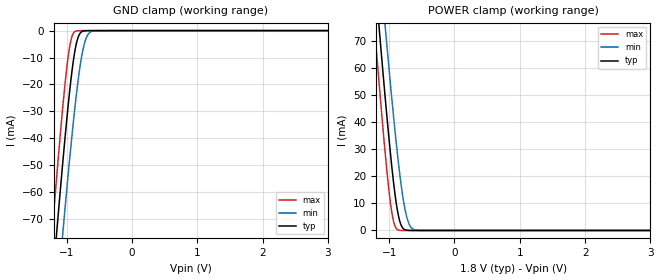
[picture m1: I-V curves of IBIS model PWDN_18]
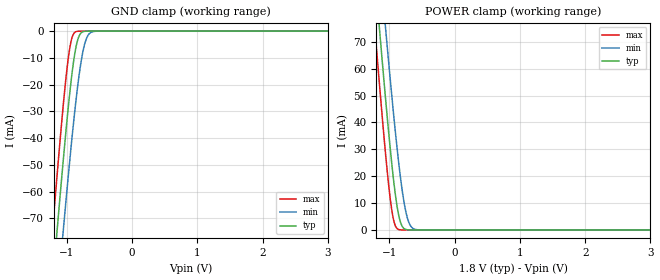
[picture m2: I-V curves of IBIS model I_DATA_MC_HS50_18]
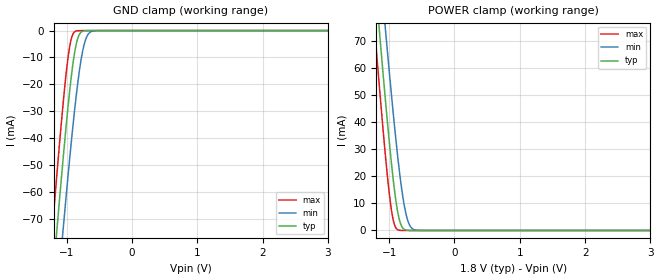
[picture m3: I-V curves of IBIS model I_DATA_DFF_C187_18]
| Texas Instruments Incorporated
| Low Power 1.8V FPD-Link (LVDS) Serializer
| Marketing part#   Voltage Range   Package-type   Temperature
| DS90C185SQE   1.71V - 1.89V   48-Pin LLP   -10 to 70C
| DS90C185SQ   1.71V - 1.89V   48-Pin LLP   -10 to 70C
| DS90C185SQX   1.71V - 1.89V   48-Pin LLP   -10 to 70C
[IBIS Ver]   4.0
[File name]   ds90c185.ibs
[File Rev]   1.0
[Date]   03/05/2012
[Source]   Model built from TISPICE simulations at:
   Texas Instruments Incorporated.
   WEBENCH DESIGN CENTER
   12500 TI Blvd
   Dallas, TX -75243
   For Support e-mail: elab_scm_ibis@list.ti.com
[Notes]   Rev 1.0: 03/05/2012
   - IBIS model generated from simulations from Spectre
   - ccomp is listed in numerical order and not by PVT case.
[Disclaimer] This product is designed as an aid for customers of Texas Instruments.
   No warranties, either expressed or implied, with respect to this third
   party software (if any) or with respect to its fitness for any
   particular purpose is claimed by Texas Instruments or the author. The
   software (if any) is provided solely on an "as is" basis. The entire
   risk as to its quality and performance is with the customer
[Copyright]   (C)Copyright 2012 Texas Instruments Incorporated.
   All rights reserved.
[Component]  DS90C185SQ
[Manufacturer]  Texas Instruments, Inc
[Package]   |48-pin LLP 6.0X6.0X0.8mm
|   typ   min   max
R_pkg   0   0   0
L_pkg   0   0   0
C_pkg   0   0   0
[Pin]   signal_name   model_name   R_pin   L_pin   C_pin
1   D9   I_DATA_DFF_C187_18
2   D10   I_DATA_DFF_C187_18
3   D11   I_DATA_DFF_C187_18
4   D12   I_DATA_DFF_C187_18
5   D13   I_DATA_DFF_C187_18
6   CLK   I_DATA_DFF_C187_18
7   D14   I_DATA_DFF_C187_18
8   D15   I_DATA_DFF_C187_18
9   D16   I_DATA_DFF_C187_18
10   D17   I_DATA_DFF_C187_18
11   D18   I_DATA_DFF_C187_18
12   D19   I_DATA_DFF_C187_18
13   VDDPLL   POWER
14   D20   I_DATA_DFF_C187_18
15   GND   GND
16   D21   I_DATA_DFF_C187_18
17   D22   I_DATA_DFF_C187_18
18   D23   I_DATA_DFF_C187_18
19   D24   I_DATA_DFF_C187_18
20   D25   I_DATA_DFF_C187_18
21   D26   I_DATA_DFF_C187_18
22   D27   I_DATA_DFF_C187_18
23   RFB   I_DATA_MC_HS50_18
24   GND   GND
25   VDDTX   POWER
26   18B_MODE   I_DATA_MC_HS50_18
27   TXOUT3P   LVDS_OUT
28   TXOUT3N   LVDS_OUT
29   TXCLKOUTP   LVDS_OUT
30   TXCLKOUTN   LVDS_OUT
31   TXOUT2P   LVDS_OUT
32   TXOUT2N   LVDS_OUT
33   TXOUT1P   LVDS_OUT
34   TXOUT1N   LVDS_OUT
35   TXOUT0P   LVDS_OUT
36   TXOUT0N   LVDS_OUT
37   PDB   PWDN_18
38   D0   I_DATA_DFF_C187_18
39   VOD_SEL   I_DATA_MC_HS50_18
40   D1   I_DATA_DFF_C187_18
41   D2   I_DATA_DFF_C187_18
42   D3   I_DATA_DFF_C187_18
43   D4   I_DATA_DFF_C187_18
44   D5   I_DATA_DFF_C187_18
45   D6   I_DATA_DFF_C187_18
46   D7   I_DATA_DFF_C187_18
47   D8   I_DATA_DFF_C187_18
48   VDD   POWER
49   DAP   GND
[Package Model] 48LLP_DS90C185
[Diff pin]  inv_pin  vdiff  tdelay_typ  tdelay_min  tdelay_max
27   28   0.0   0.0s   0.0s   0.0s
29   30   0.0   0.0s   0.0s   0.0s
31   32   0.0   0.0s   0.0s   0.0s
33   34   0.0   0.0s   0.0s   0.0s
35   36   0.0   0.0s   0.0s   0.0s
[Define Package Model]  48LLP_DS90C185
| AD# DS90C1855SQ-01 RevA at 6GHz
[Manufacturer]  Unknown
[OEM]  Unknown
[Description]  None
[Number Of Pins]  48
[Pin Numbers]
|Pin Num   Terminal Name
1   | L1:1
2   | L2:2
3   | L3:3
4   | L4:4
5   | L5:5
6   | L6:6
7   | L7:7
8   | L8:8
9   | L9:9
10   | L10:10
11   | L11:11
12   | L12:12
13   | L13:13
14   | L14:14
15   | L15:15
16   | L16:16
17   | L17:17
18   | L18:18
19   | L19:19
20   | L20:20
21   | L21:21
22   | L22:22
23   | L23:23
24   | L24:24
25   | L25:25
26   | L26:26
27   | L27:27
28   | L28:28
29   | L29:29
30   | L30:30
31   | L31:31
32   | L32:32
33   | L33:33
34   | L34:34
35   | L35:35
36   | L36:36
37   | L37:37
38   | L38:38
39   | L39:39
40   | L40:40
41   | L41:41
42   | L42:42
43   | L43:43
44   | L44:44
45   | L45:45
46   | L46:W50
47   | L47:47
48   | L48:48
[Model Data]
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[End Model Data]
[End Package Model]
| Models and submodels in the file (4): PWDN_18 (Input), I_DATA_MC_HS50_18 (Input), I_DATA_DFF_C187_18 (Input), LVDS_OUT (Output)
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[Model]   PWDN_18
Model_type   Input
Vinl = 0.63V
Vinh = 1.17V
|   typ   min   max
|   (nom)   (weak)   (fast)
C_comp   0.5928pF   0.5928pF   0.5928pF
[Voltage Range]   1.800V   1.710V   1.890V
[Temperature Range]   25.0   105.0   -40.0
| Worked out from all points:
|   GND clamp passes 1 mA (typ) near -0.79 V on its own axis
|   POWER clamp passes 1 mA (typ) near -0.79 V on its own axis
[GND Clamp]
|   Voltage   I(typ)   I(min)   I(max)
-1.8V     -270.9mA   -291mA     -255.6mA
-1.228V   -97.1mA    -122.7mA   -76.77mA
-1.201V   -89.21mA   -115mA     -68.71mA
-1.147V   -73.63mA   -99.73mA   -52.87mA
-1.055V   -48.06mA   -74.39mA   -27.51mA
-957.6mV  -23.54mA   -48.82mA   -6.663mA
-871.2mV  -7.328mA   -28.21mA   -335.2uA
-811.8mV  -1.781mA   -16.28mA   -25.67uA
-741.6mV  -161.6uA   -6.205mA   -6.921uA
-682.2mV  -20.1uA    -1.83mA    -5.854uA
-601.2mV  -4.02uA    -199.2uA   -5.127uA
3.595V    6.712uA    3.483uA    12.03uA
[POWER Clamp]
|   Voltage   I(typ)   I(min)   I(max)
-1.8V     270.2mA    290.2mA    254.8mA
-1.228V   96.77mA    122.3mA    76.49mA
-1.201V   88.9mA     114.6mA    68.45mA
-1.147V   73.36mA    99.39mA    52.65mA
-1.055V   47.86mA    74.11mA    27.37mA
-957.6mV  23.41mA    48.61mA    6.6mA
-871.2mV  7.262mA    28.06mA    325.8uA
-811.8mV  1.758mA    16.17mA    20.65uA
-741.6mV  156.5uA    6.146mA    2.661uA
-682.2mV  17.07uA    1.807mA    2.011uA
-601.2mV  1.608uA    195uA      1.824uA
3.595V    0A         0A         0A
[Model]   I_DATA_MC_HS50_18
Model_type   Input
Vinl = 0.63V
Vinh = 1.17V
|   typ   min   max
|   (nom)   (weak)   (fast)
C_comp   0.5928pF   0.5928pF   0.5928pF
[Voltage Range]   1.800V   1.710V   1.890V
[Temperature Range]   25.0   105.0   -40.0
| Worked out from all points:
|   GND clamp passes 1 mA (typ) near -0.79 V on its own axis
|   POWER clamp passes 1 mA (typ) near -0.79 V on its own axis
[GND Clamp]
|   Voltage   I(typ)   I(min)   I(max)
-1.8V     -271mA     -291mA     -255.6mA
-1.228V   -97.13mA   -122.7mA   -76.8mA
-1.201V   -89.24mA   -115mA     -68.74mA
-1.147V   -73.66mA   -99.76mA   -52.9mA
-1.055V   -48.09mA   -74.42mA   -27.54mA
-957.6mV  -23.57mA   -48.85mA   -6.691mA
-871.2mV  -7.355mA   -28.24mA   -349uA
-811.8mV  -1.796mA   -16.31mA   -35.11uA
-741.6mV  -166.7uA   -6.23mA    -13.16uA
-682.2mV  -22.73uA   -1.842mA   -9.797uA
-601.2mV  -4.882uA   -201.7uA   -6.456uA
3.595V    0A         0A         0A
[POWER Clamp]
|   Voltage   I(typ)   I(min)   I(max)
-1.8V     270.2mA    290.2mA    254.9mA
-1.228V   96.77mA    122.3mA    76.49mA
-1.201V   88.91mA    114.6mA    68.45mA
-1.147V   73.37mA    99.4mA     52.66mA
-1.055V   47.86mA    74.12mA    27.37mA
-957.6mV  23.41mA    48.61mA    6.602mA
-871.2mV  7.263mA    28.06mA    324uA
-811.8mV  1.758mA    16.17mA    18.49uA
-741.6mV  155.5uA    6.146mA    576.2nA
-682.2mV  16.1uA     1.807mA    26.76nA
-601.2mV  704.2nA    194.6uA    0A
3.595V    0A         0A         0A
[Model]   I_DATA_DFF_C187_18
Model_type   Input
Vinl = 0.63V
Vinh = 1.17V
|   typ   min   max
|   (nom)   (weak)   (fast)
C_comp   0.5928pF   0.5928pF   0.5928pF
[Voltage Range]   1.800V   1.710V   1.890V
[Temperature Range]   25.0   105.0   -40.0
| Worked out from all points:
|   GND clamp passes 1 mA (typ) near -0.79 V on its own axis
|   POWER clamp passes 1 mA (typ) near -0.79 V on its own axis
[GND Clamp]
|   Voltage   I(typ)   I(min)   I(max)
-1.8V     -271mA     -291mA     -255.6mA
-1.228V   -97.13mA   -122.7mA   -76.8mA
-1.201V   -89.24mA   -115mA     -68.74mA
-1.147V   -73.66mA   -99.76mA   -52.9mA
-1.055V   -48.09mA   -74.42mA   -27.54mA
-957.6mV  -23.57mA   -48.85mA   -6.691mA
-871.2mV  -7.355mA   -28.24mA   -349uA
-811.8mV  -1.796mA   -16.31mA   -35.11uA
-741.6mV  -166.7uA   -6.23mA    -13.16uA
-682.2mV  -22.73uA   -1.842mA   -9.797uA
-601.2mV  -4.882uA   -201.7uA   -6.455uA
3.595V    0A         0A         0A
[POWER Clamp]
|   Voltage   I(typ)   I(min)   I(max)
-1.8V     270.2mA    290.2mA    254.9mA
-1.228V   96.77mA    122.3mA    76.49mA
-1.201V   88.91mA    114.6mA    68.45mA
-1.147V   73.37mA    99.4mA     52.66mA
-1.055V   47.86mA    74.12mA    27.37mA
-957.6mV  23.41mA    48.61mA    6.602mA
-871.2mV  7.263mA    28.06mA    324uA
-811.8mV  1.758mA    16.17mA    18.49uA
-741.6mV  155.5uA    6.146mA    576.2nA
-682.2mV  16.1uA     1.807mA    26.76nA
-601.2mV  704.2nA    194.6uA    0A
3.595V    0A         0A         0A
